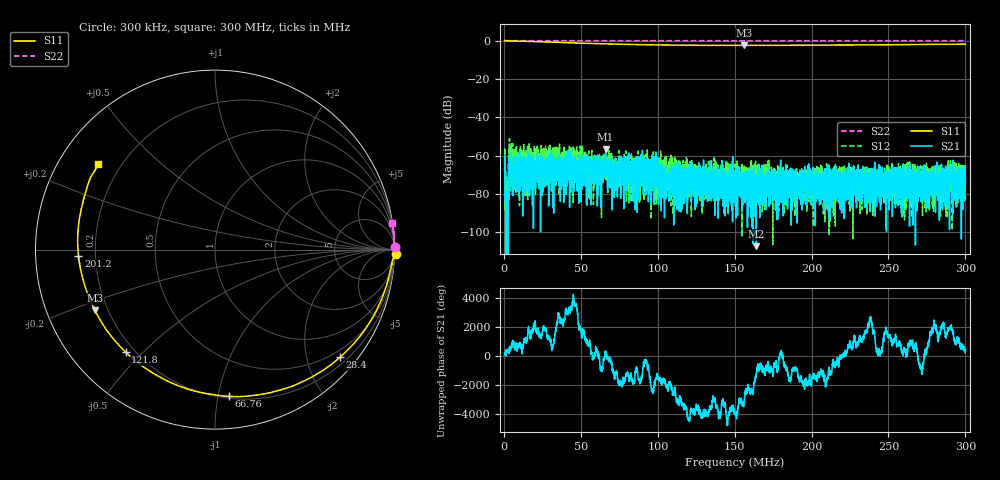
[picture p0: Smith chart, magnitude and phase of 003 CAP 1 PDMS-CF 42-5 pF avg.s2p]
!  26/06/2025  14:58:55
! Ref Plane: 0.000 mm
# MHZ S MA R  50
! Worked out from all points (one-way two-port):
!   4001 points, 300 kHz to 300 MHz, reference 50 ohm
!   highest |S21| = -56.52 dB at 66.01 MHz (marker M1); lowest = -107.3 dB at 164 MHz (marker M2)
!   lowest |S11| = -2.5 dB at 155.9 MHz (marker M3), VSWR 6.97, Z = 7.57 - j11.7 ohm
!   |S11| at or under -10 dB: nowhere
!   |S22| runs from 0.0 to 0.1 dB; largest |S21 - S12| = 0.0034
!   S11 on the Smith chart (normalised r, x): 300 kHz: -27, -72; 28.4 MHz: 0.35, -2.66; 66.76 MHz: 0.21, -1.08; 121.8 MHz: 0.17, -0.44; 201.2 MHz: 0.14, -0.02; 300 MHz: 0.12, +0.32
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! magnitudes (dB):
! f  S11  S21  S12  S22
! 300 kHz  0.1  -68.6  -64.0  0.0
! 2.023 MHz  -0.1  -86.0  -73.4  0.0
! 4.346 MHz  -0.2  -67.6  -57.6  0.0
! 13.79 MHz  -0.3  -74.5  -61.4  0.0
! 28.4 MHz  -0.7  -65.4  -64.4  0.0
! 50.28 MHz  -1.3  -70.9  -66.4  0.0
! 62.04 MHz  -1.6  -70.1  -63.0  0.0
! 66.01 MHz  -1.7  -56.5  -72.5  0.0
! 66.76 MHz  -1.7  -66.6  -65.2  0.0
! 77.18 MHz  -1.9  -65.9  -63.1  0.0
! 90.22 MHz  -2.1  -63.0  -67.2  0.0
! 100.3 MHz  -2.2  -82.7  -74.6  0.0
! 116.4 MHz  -2.4  -67.5  -62.4  0.0
! 121.8 MHz  -2.4  -63.0  -67.3  0.0
! 150.2 MHz  -2.5  -83.7  -72.1  0.0
! 155.9 MHz  -2.5  -72.4  -74.4  0.0
! 164 MHz  -2.5  -107.3  -71.6  0.0
! 183.4 MHz  -2.4  -85.9  -81.7  0.0
! 200.1 MHz  -2.4  -68.2  -70.9  0.0
! 201.2 MHz  -2.4  -73.2  -97.1  0.0
! 250.1 MHz  -2.2  -82.4  -70.1  0.0
! 300 MHz  -1.9  -74.2  -73.3  0.0
